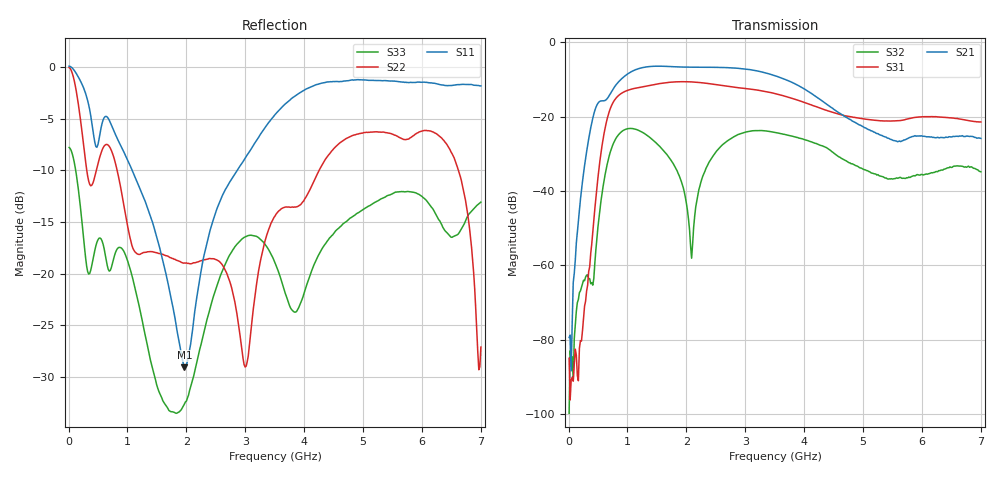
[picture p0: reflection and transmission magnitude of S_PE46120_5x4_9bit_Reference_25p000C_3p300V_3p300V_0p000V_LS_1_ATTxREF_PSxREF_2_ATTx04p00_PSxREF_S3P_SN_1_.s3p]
! Device ID: PE46120_5x4_9bit_Reference
! Device ID: PE46120_5x4_9bit_Reference
! File Path: z:\PE46120_5x4_9bit_Reference\MPAC_Yi\new_12port\25p000C\3p300\LS_1_ATTxREF_PSxREF_2_ATTx04p00_PSxREF\PE46120_5x4_9bit_Reference_25p000C_3p300V_3p300V_0p000V_LS_1_ATTxREF_PSxREF_2_ATTx04p00_PSxREF_S3P_SN_1_.s3p
! Serial: 1
! Lot:
! Temp: 25.000C
! VDD: 3.300
! VSS: 0.000
! Control_Hi: 3.300
! Control_Lo: 0.000
! Logic State: LS_1_ATTxREF_PSxREF_2_ATTx04p00_PSxREF
! Port 1: RFin
! Port 2: RFout1
! Port 3: RFout2
! ThroughPath:1-3
! IDD: -0.0005393673
! ISS: 0
! Comment:
#  Hz  S  RI  R  50
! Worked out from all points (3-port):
!   401 points, 10 MHz to 7 GHz, reference 50 ohm
!   strongest paths, dB at 10 MHz, 1.758 GHz, 3.505 GHz, 5.253 GHz, 7 GHz:
!     S21: -79.4, -6.6, -9.0, -24.6, -25.9
!     S31: -85.0, -10.7, -13.8, -21.1, -21.4
!     S32: -99.7, -32.2, -24.2, -35.6, -34.8
!   lowest |S11| = -29.0 dB at 1.967 GHz (marker M1), VSWR 1.07, Z = 52.8 + j2.36 ohm
!   |S11| at or under -10 dB: 1.079 GHz to 2.863 GHz (1.784 GHz wide, 90.5 % of centre)
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1e7  1.001 -0.115  4.53e-05 -0.000105  -1.43e-05 1.41e-05
     -2.85e-06 -0.000107  0.9868 -0.0965  -1.13e-06 -2.38e-05
     5.54e-05 -1.11e-05  7.01e-06 7.54e-06  0.4057 -0.0383
2.37175e8  -0.4764 -0.6603  -0.0122 -0.0053  5.92e-05 0.000164
           -0.0123 -0.0055  -0.2982 -0.3552  -0.000108 0.000578
           5.37e-05 0.000122  -0.000153 0.000548  -0.1016 -0.1336
4.6435e8  -0.4061 -0.0666  -0.0601 0.1164  0.00758 0.00267
          -0.0607 0.118  0.1371 0.2774  -0.00109 0.00121
          0.0076 0.00264  -0.00113 0.00117  0.0782 0.1117
9.187e8  -0.3044 0.2575  0.3267 -0.0185  -0.0991 0.1818
         0.3307 -0.0189  -0.04 -0.2281  -0.0472 0.0426
         -0.1004 0.1843  -0.0478 0.0431  0.0777 -0.1055
1.9672e9  0.0274 0.0223  -0.3832 0.2487  -0.1648 -0.2392
          -0.3876 0.2522  -0.0946 0.0611  0.000134 0.0092
          -0.1673 -0.2417  0.000306 0.00953  -0.000184 0.0234
2.089525e9  0.047 -0.0154  -0.277 0.3616  -0.2388 -0.1614
            -0.2798 0.3663  -0.0607 0.0939  0.00124 -0.000414
            -0.2423 -0.1632  0.00105 -0.000676  -0.00294 0.0293
2.49145e9  0.0274 -0.1936  0.2028 0.4058  -0.2296 0.1348
           0.2055 0.4104  0.0851 0.0806  -0.0279 0.016
           -0.2325 0.137  -0.0283 0.0162  0.00545 0.0827
3.505e9  -0.4337 -0.3957  -0.0902 -0.3374  0.1989 0.0306
         -0.0914 -0.3418  0.0623 0.1793  0.00723 -0.06
         0.2013 0.0305  0.00689 -0.061  0.1085 -0.0307
6.26605e9  -0.3685 0.7396  0.0393 -0.0331  -0.00729 0.0973
           0.0401 -0.0341  0.4574 -0.1066  -0.0184 -0.00172
           -0.00725 0.0988  -0.018 -0.00203  0.1849 -0.0216
7e9  -0.1131 0.8008  -0.0289 -0.0407  0.0748 0.0361
     -0.0298 -0.0413  -0.0391 0.0205  0.0159 0.00682
     0.0767 0.036  0.0163 0.0079  0.1724 0.1395
